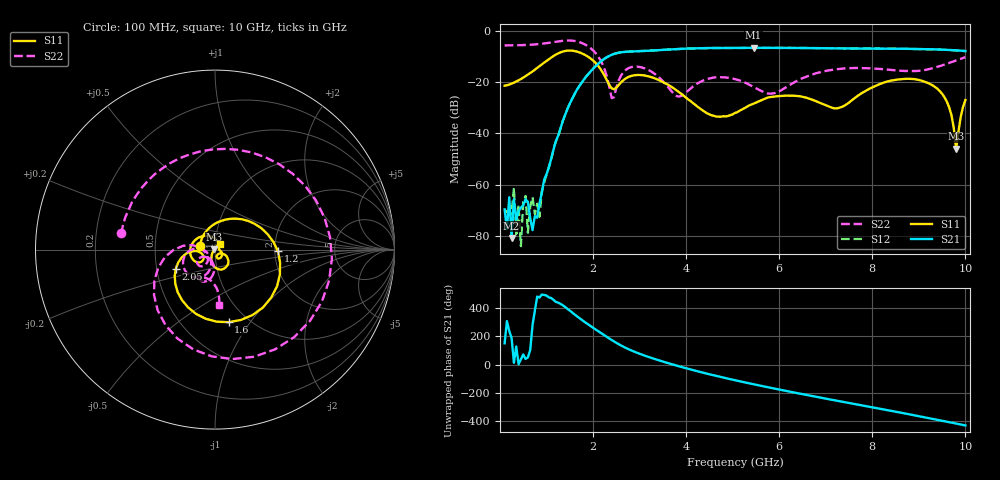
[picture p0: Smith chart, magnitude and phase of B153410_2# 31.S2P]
!  2-Port S-parameters saved by WinCal
! VAR MeasName=S-Parameters (CALIBRATED_DATA) read from VNA (N5245A)
! VAR MeasDate=2016-12-23 10:00:55
! VAR NAME=B153410_2# 31
! VAR FILENAME=B153410_2# 31.S2P
! VAR DATE=2016-12-23 10:00:55
! VAR PHYS_PORTS=1,2
# Hz S DB R 50
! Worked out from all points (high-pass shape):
!   199 points, 100 MHz to 10 GHz, reference 50 ohm
!   highest |S21| = -6.44 dB at 5.45 GHz (marker M1); lowest = -81.0 dB at 250 MHz (marker M2)
!   |S21| within 3 dB of the highest: 2.37 GHz to end of sweep
!   lowest |S11| = -45.9 dB at 9.8 GHz (marker M3), VSWR 1.01, Z = 49.5 + j0.102 ohm
!   |S11| at or under -10 dB: start of sweep to 1.124 GHz; 1.897 GHz to end of sweep
!   |S22| runs from -26.1 to -3.6 dB; largest |S21 - S12| = 0.0033
!   S11 on the Smith chart (normalised r, x): 100 MHz: 0.85, +0.04; 1.2 GHz: 2.08, -0.05; 1.6 GHz: 0.82, -0.80; 2.05 GHz: 0.63, -0.14; 10 GHz: 1.06, +0.07
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1e8  -21.27 165.0  -69.71 150.5  -69.80 -50.8  -5.52 170.2
2e8  -20.85 150.0  -64.99 -122.9  -70.88 168.2  -5.50 160.4
2.5e8  -20.48 142.2  -80.97 -170.4  -71.32 81.2  -5.51 155.3
3e8  -20.12 134.8  -65.72 13.3  -61.34 139.9  -5.47 150.2
3.5e8  -19.65 127.2  -73.68 128.4  -79.44 -66.9  -5.47 145.0
5.5e8  -17.56 98.6  -65.76 40.2  -64.48 36.3  -5.37 123.1
6e8  -16.95 91.6  -66.78 51.1  -78.90 -10.7  -5.31 117.2
7e8  -15.72 77.6  -77.86 -80.7  -64.95 15.7  -5.21 104.8
8.5e8  -13.66 56.0  -67.33 114.6  -72.64 -180.0  -4.98 84.4
1.2e9  -9.09 -1.6  -43.01 83.4  -43.24 83.3  -4.07 25.8
1.6e9  -7.71 -79.3  -24.64 -3.7  -24.66 -3.7  -3.76 -59.0
1.75e9  -8.55 -106.4  -20.24 -41.7  -20.25 -41.7  -4.51 -91.8
2.05e9  -12.30 -154.2  -13.74 -110.3  -13.73 -110.2  -8.42 -152.9
2.4e9  -22.30 -163.6  -9.20 174.1  -9.19 174.0  -26.14 -165.6
3.4e9  -18.95 143.3  -7.39 31.7  -7.38 31.7  -17.77 179.9
5.05e9  -31.95 -5.8  -6.48 -110.6  -6.49 -110.4  -18.71 -148.4
5.45e9  -28.33 -21.5  -6.44 -139.0  -6.46 -139.0  -21.81 -150.4
6.7e9  -26.70 -76.2  -6.56 138.2  -6.56 138.2  -16.97 -94.9
8.35e9  -19.53 -45.8  -6.82 36.4  -6.81 36.6  -15.03 -115.7
9.4e9  -22.49 -103.6  -7.13 -30.6  -7.12 -30.5  -13.91 -89.7
9.8e9  -45.95 168.3  -7.47 -57.0  -7.48 -56.9  -11.38 -85.2
1e10  -26.91 48.6  -7.72 -70.5  -7.76 -70.2  -10.11 -85.8
